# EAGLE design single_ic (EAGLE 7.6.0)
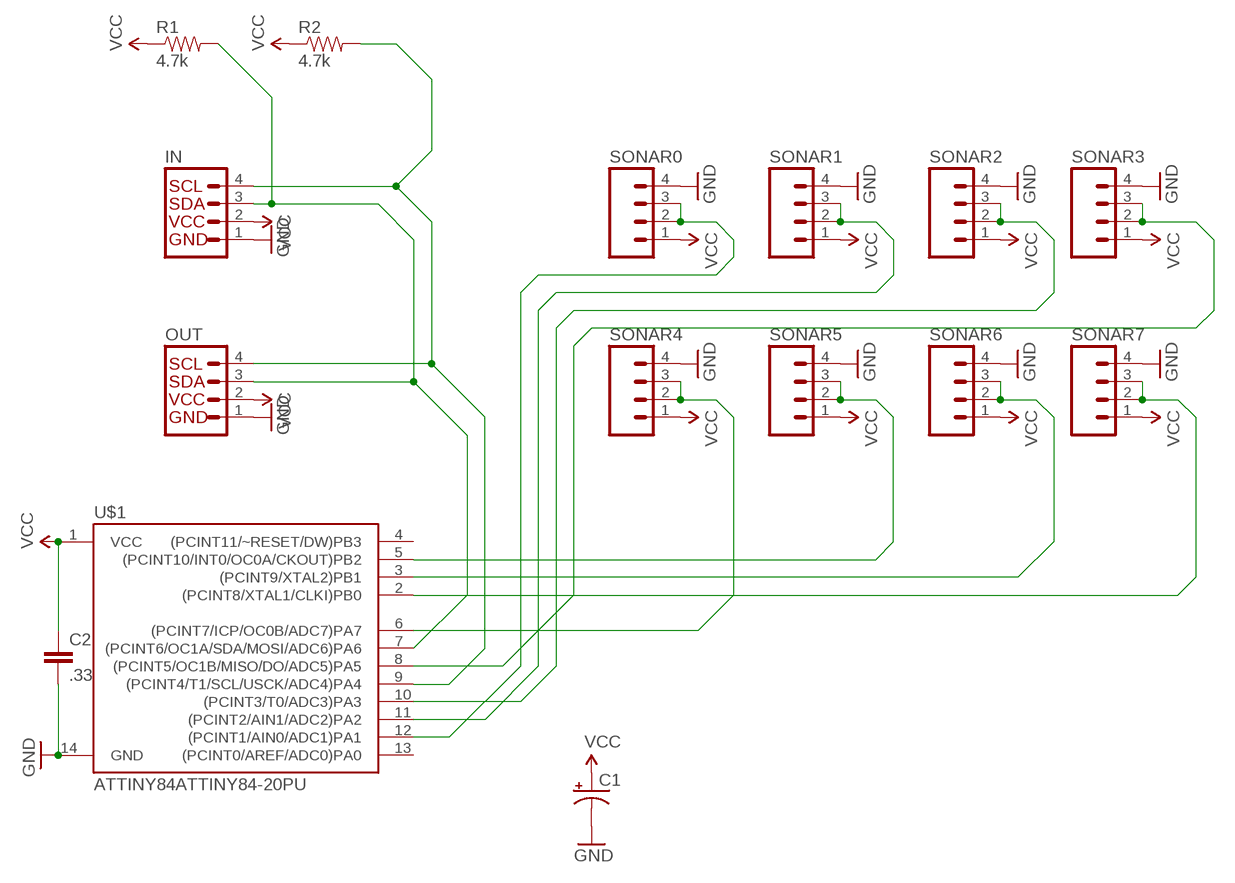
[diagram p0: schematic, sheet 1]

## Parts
C1  100UF-25V-20%(PTH)  [CPOL-RADIAL-100UF-25V]
C2  .33  CAPPTH1  [CAP-PTH-5MM]
IN  I2C_STANDARD  [1X04]
OUT  I2C_STANDARD  [1X04]
R1  4.7k  RESISTORKIT  [AXIAL-0.3-KIT]
R2  4.7k  RESISTORKIT  [AXIAL-0.3-KIT]
SONAR0  M04NO_SILK_ALL_ROUND  [1X04_NO_SILK_ALL_ROUND]
SONAR1  M04NO_SILK_ALL_ROUND  [1X04_NO_SILK_ALL_ROUND]
SONAR2  M04NO_SILK_ALL_ROUND  [1X04_NO_SILK_ALL_ROUND]
SONAR3  M04NO_SILK_ALL_ROUND  [1X04_NO_SILK_ALL_ROUND]
SONAR4  M04NO_SILK_ALL_ROUND  [1X04_NO_SILK_ALL_ROUND]
SONAR5  M04NO_SILK_ALL_ROUND  [1X04_NO_SILK_ALL_ROUND]
SONAR6  M04NO_SILK_ALL_ROUND  [1X04_NO_SILK_ALL_ROUND]
SONAR7  M04NO_SILK_ALL_ROUND  [1X04_NO_SILK_ALL_ROUND]
U$1  ATTINY84ATTINY84-20PU  [DIL14]

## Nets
GND: C1.2(-) C2.2 IN.1 OUT.1 SONAR0.4 SONAR1.4 SONAR2.4 SONAR3.4 SONAR4.4 SONAR5.4 SONAR6.4 SONAR7.4 U$1.14(GND)
N$1: IN.4 OUT.4 R2.P$2 U$1.9((PCINT4/T1/SCL/USCK/ADC4)PA4)
N$2: SONAR6.2 SONAR6.3 U$1.3((PCINT9/XTAL2)PB1)
N$3: IN.3 OUT.3 R1.P$2 U$1.7((PCINT6/OC1A/SDA/MOSI/ADC6)PA6)
N$5: SONAR0.2 SONAR0.3 U$1.12((PCINT1/AIN0/ADC1)PA1)
N$6: SONAR1.2 SONAR1.3 U$1.11((PCINT2/AIN1/ADC2)PA2)
N$7: SONAR2.2 SONAR2.3 U$1.10((PCINT3/T0/ADC3)PA3)
N$8: SONAR3.2 SONAR3.3 U$1.8((PCINT5/OC1B/MISO/DO/ADC5)PA5)
N$9: SONAR4.2 SONAR4.3 U$1.6((PCINT7/ICP/OC0B/ADC7)PA7)
N$10: SONAR5.2 SONAR5.3 U$1.5((PCINT10/INT0/OC0A/CKOUT)PB2)
N$12: SONAR7.2 SONAR7.3 U$1.2((PCINT8/XTAL1/CLKI)PB0)
VCC: C1.1(+) C2.1 IN.2 OUT.2 R1.P$1 R2.P$1 SONAR0.1 SONAR1.1 SONAR2.1 SONAR3.1 SONAR4.1 SONAR5.1 SONAR6.1 SONAR7.1 U$1.1(VCC)
Unconnected: U$1.4((PCINT11/~RESET/DW)PB3) U$1.13((PCINT0/AREF/ADC0)PA0)

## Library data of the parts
C1 = SparkFun-Capacitors:100UF-25V-20%(PTH): CAP-08439; PROD_ID: CAP-08439
C2 = SparkFun-Capacitors:CAP: Capacitor
IN OUT = SparkFun-Connectors:I2C_STANDARD: SparkFun has standardized on a pinout for all I2C based sensor breakouts. This pinout allows I2C boards to be plugged directly into the headers on Arduino Uno compatible boards, and to be daisy chained easily.
R1 R2 = SparkFun-Resistors:RESISTOR: Resistor
SONAR0 SONAR1-SONAR7 = SparkFun-Connectors:M04: Header 4 Standard 4-pin 0.1" header. Use with straight break away headers (SKU : PRT-00116), right angle break away headers (PRT-00553), swiss pins (PRT-00743), machine pins (PRT-00117), and female headers (PRT-00115). Molex polarized connector foot print use with SKU : PRT-08231 with associated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; PROD_ID: CONN-09696
U$1 = SparkFun-DigitalIC:ATTINY84: Atmel 14-pin 2/4/8kB flash uC

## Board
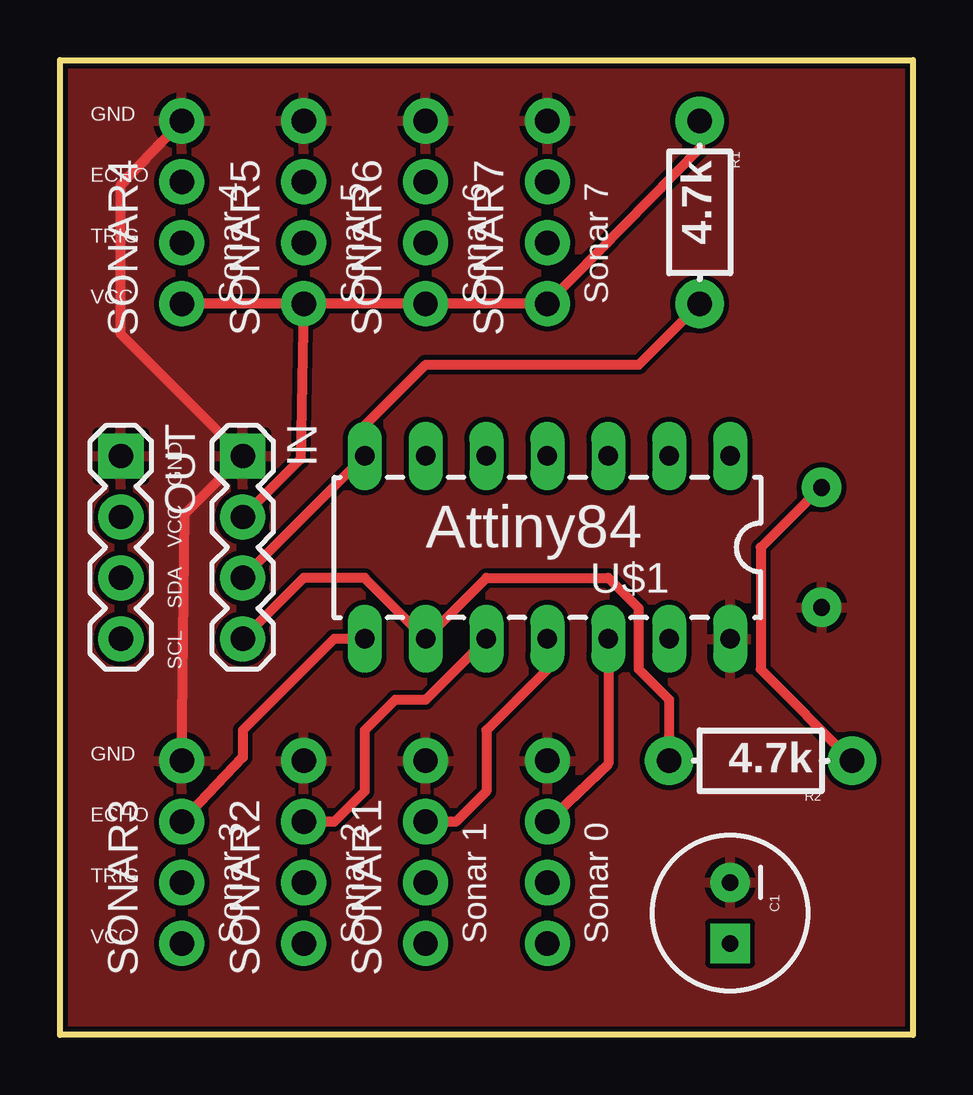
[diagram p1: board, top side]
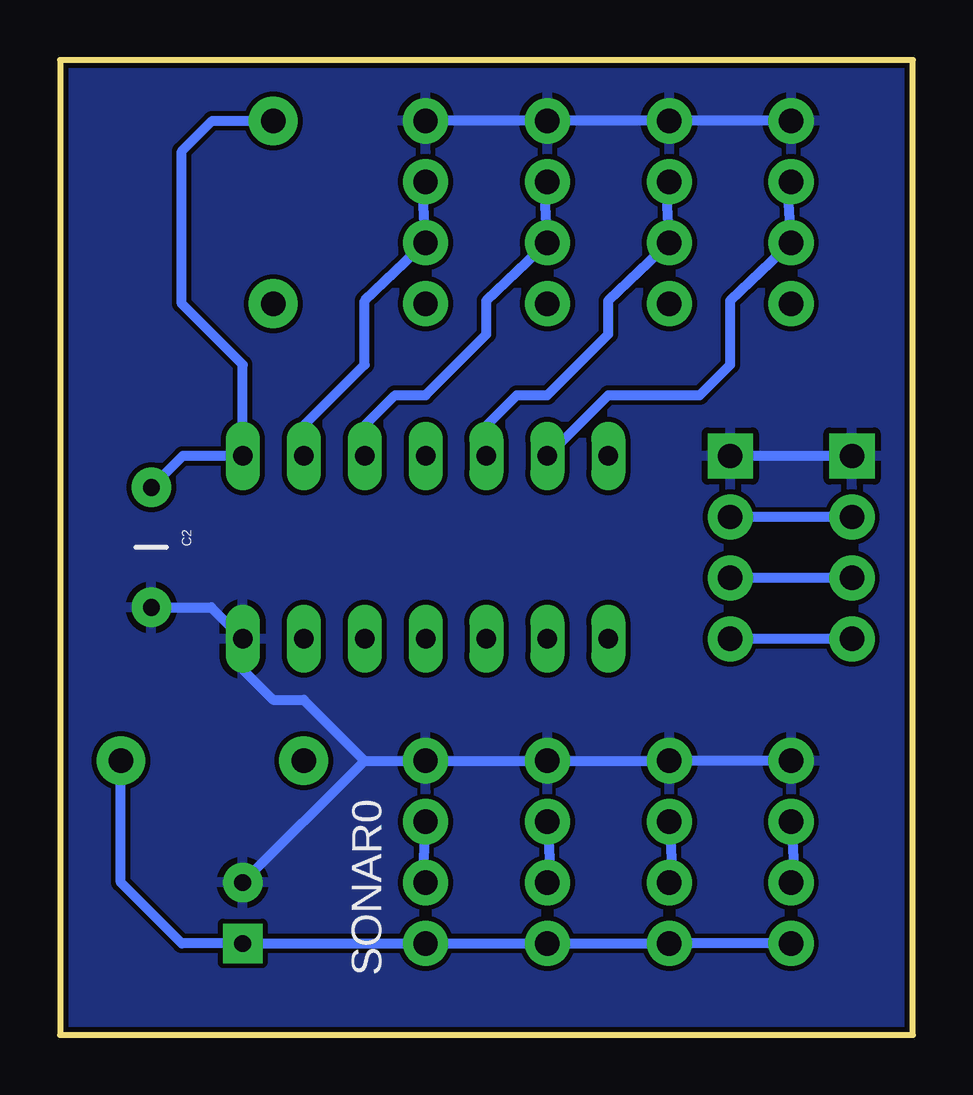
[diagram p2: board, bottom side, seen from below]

Size 35.56 x 40.64 mm. Coordinates in mm from the lower left corner, seen from the top.
Outline: 0,0 0,40.64 35.56,40.64 35.56,0 0,0
Copper layers (1*16): Top 0.035mm / dielectric 1.5mm / Bottom 0.035mm
Design rules "SparkFun": minimum track width 8mil, minimum drill 20mil, track to track 8mil, track to pad 8mil, pad to pad 8mil, via to via 8mil, smd to smd 8mil, copper to edge 8mil, drill to drill 8mil, minimum pad ring 12mil, minimum via ring 10mil, stop-mask expansion 4mil, vias tented up to drill 20mil, thermal gap 10mil

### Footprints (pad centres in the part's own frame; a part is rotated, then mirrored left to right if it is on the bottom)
CPOL-RADIAL-100UF-25V = drill 0.7 pad 1.651 square: 1 1.27,0 | drill 0.7 pad 1.651: 2 -1.27,0
CAP-PTH-5MM = drill 0.7 pad 1.651: 1 -2.5,0; 2 2.5,0
1X04 = drill 1.016 pad 1.88 square: 1 0,0 | drill 1.016 pad 1.88: 2 2.54,0; 3 5.08,0; 4 7.62,0
AXIAL-0.3-KIT = drill 1.016 pad 2.032: P$1 -3.81,0; P$2 3.81,0
1X04_NO_SILK_ALL_ROUND = drill 1.016 pad 1.88: 1 0,0; 2 2.54,0; 3 5.08,0; 4 7.62,0
DIL14 = drill 0.813 long: 1 -8.89,-3.81; 2 -6.35,-3.81; 3 -3.81,-3.81; 4 -1.27,-3.81; 5 1.27,-3.81; 6 3.81,-3.81; 7 6.35,-3.81; 8 6.35,3.81; 9 3.81,3.81; 10 1.27,3.81; 11 -1.27,3.81; 12 -3.81,3.81; 13 -6.35,3.81; 14 -8.89,3.81

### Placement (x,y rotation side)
C1  27.94,5.08 270 top
C2  31.75,20.32 270 bottom
IN  7.62,24.13 270 top
OUT  2.54,24.13 270 top
R1  26.67,34.29 270 top
R2  29.21,11.43 180 top
SONAR0  20.32,3.81 90 bottom
SONAR1  15.24,3.81 90 top
SONAR2  10.16,3.81 90 top
SONAR3  5.08,3.81 90 top
SONAR4  5.08,30.48 90 top
SONAR5  10.16,30.48 90 top
SONAR6  15.24,30.48 90 top
SONAR7  20.32,30.48 90 top
U$1  19.05,20.32 180 top

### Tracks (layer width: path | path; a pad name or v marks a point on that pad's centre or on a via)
GND
  Top 0.406: SONAR4.4 2.54,35.43 2.54,29.21 IN.1 5.21,21.72 SONAR3.4
  Bottom 0.406: SONAR4.4 SONAR5.4 SONAR6.4 SONAR7.4 | C2.2 29.25,17.82 U$1.14 27.94,15.24 26.67,13.97 25.4,13.97 22.86,11.43 | C1.2 22.86,11.43 | 22.86,11.43 SONAR0.4 SONAR1.4 SONAR2.4 SONAR3.4 | OUT.1 IN.1
  pour Top: 0,0 0,40.64 35.56,40.64 35.56,0
  pour Bottom: 0,0 0,40.64 35.56,40.64 35.56,0
N$1
  Top 0.406: R2.P$2 25.4,13.97 24.13,15.24 24.13,17.78 22.86,19.05 17.78,19.05 U$1.9 12.7,19.05 10.16,19.05 IN.4
  Bottom 0.406: OUT.4 IN.4
N$2
  Bottom 0.406: U$1.3 22.86,25.4 21.59,26.67 20.32,26.67 17.78,29.21 17.78,30.61 SONAR6.2 15.37,35.31 SONAR6.3
N$3
  Top 0.406: IN.3 U$1.7 12.7,25.4 15.24,27.94 24.13,27.94 R1.P$2
  Bottom 0.406: OUT.3 IN.3
N$5
  Top 0.406: U$1.12 22.86,11.3 SONAR0.3
  Bottom 0.406: SONAR0.3 20.45,6.6 SONAR0.2
N$6
  Top 0.406: U$1.11 20.32,15.24 17.78,12.7 17.78,10.16 16.51,8.89 SONAR1.3
  Bottom 0.406: SONAR1.3 15.11,6.6 SONAR1.2
N$7
  Top 0.406: U$1.10 15.24,13.97 13.97,13.97 12.7,12.7 12.7,10.16 11.43,8.89 SONAR2.3
  Bottom 0.406: SONAR2.3 10.03,6.6 SONAR2.2
N$8
  Top 0.406: U$1.8 11.43,16.51 7.62,12.7 7.62,11.56 SONAR3.3
  Bottom 0.406: SONAR3.3 4.95,6.6 SONAR3.2
N$9
  Bottom 0.406: U$1.6 12.7,26.67 8.89,26.67 7.62,27.94 7.62,30.61 SONAR4.2 5.21,35.31 SONAR4.3
N$10
  Bottom 0.406: U$1.5 17.78,25.4 16.51,26.67 15.24,26.67 12.7,29.21 12.7,30.61 SONAR5.2 10.29,35.31 SONAR5.3
N$12
  Bottom 0.406: U$1.2 25.4,25.4 22.86,27.94 22.86,30.61 SONAR7.2 20.45,35.31 SONAR7.3
VCC
  Top 0.406: R1.P$1 26.67,36.96 SONAR7.1 SONAR6.1 SONAR5.1 | SONAR5.1 SONAR4.1 | SONAR5.1 10.03,24 IN.2 | C2.1 31.71,22.82 29.21,20.32 29.21,15.24 R2.P$1
  Bottom 0.406: C2.1 30.44,24.13 U$1.1 27.94,27.94 30.48,30.48 30.48,36.83 29.21,38.1 R1.P$1 | R2.P$1 33.02,6.35 30.48,3.81 C1.1 SONAR0.1 SONAR1.1 SONAR2.1 SONAR3.1 | OUT.2 IN.2

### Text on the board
tPlace: GND | ECHO | TRIG | VCC | Sonar 4 | Sonar 5 | Sonar 6 | Sonar 7 | GND | VCC | Attiny84 | SDA | SCL | GND | ECHO | TRIG | VCC | Sonar 3 | Sonar 2 | Sonar 1 | Sonar 0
